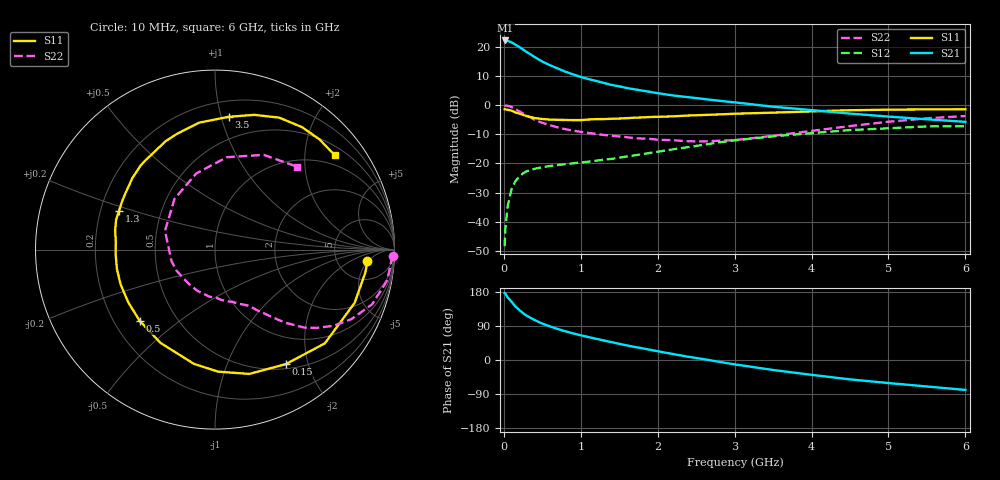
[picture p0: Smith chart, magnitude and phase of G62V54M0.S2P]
! SIEMENS Small Signal Semiconductors
! BFG193
! Si NPN RF Bipolar Junction Transistor in SOT223
! VCE = 2.5 V  IC = 4 mA
! Common Emitter S-Parameters:  August  1996
# GHz  S  MA  R  50
!  f  S11  S21  S12  S22
! GHz  MAG  ANG  MAG  ANG  MAG  ANG  MAG  ANG
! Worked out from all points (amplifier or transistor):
!   36 points, 10 MHz to 6 GHz, reference 50 ohm
!   highest |S21| = 22.2 dB at 20 MHz (marker M1)
!   |S21| within 3 dB of that: start of sweep to 243.1 MHz
!   unconditionally stable (mu >= 1): 1.209 GHz to 2.622 GHz
!   at 250 MHz: K = 0.29, MSG = 21.2 dB, |S12| = -23.4 dB
!   at 1.4 GHz: K = 1.09, MAG = 10.9 dB, |S12| = -18.4 dB
!   at 6 GHz: K = 0.92, MSG = 0.7 dB, |S12| = -7.2 dB
!   S11 on the Smith chart (normalised r, x): 10 MHz: 10, -5; 150 MHz: 0.56, -1.65; 500 MHz: 0.31, -0.37; 1.3 GHz: 0.28, +0.18; 3.5 GHz: 0.32, +1.06; 6 GHz: 0.72, +2.71
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0.01  0.851 -4.3  12.84 176.9  0.0038 89.4  0.9933 -2.0
0.02  0.8475 -8.6  12.9 175.1  0.0075 86.8  0.9831 -4.1
0.05  0.8326 -20.9  12.67 165.3  0.0186 78.9  0.9751 -10.1
0.1  0.8046 -40.5  11.95 153.8  0.036 70.3  0.927 -19.2
0.15  0.7502 -58.3  10.92 141.2  0.0493 60.3  0.8531 -27.0
0.2  0.7185 -74.6  9.979 132.2  0.0592 54.3  0.7855 -32.7
0.25  0.6801 -88.6  9 123.5  0.0676 48.5  0.7151 -37.6
0.3  0.6473 -100.5  8.134 116.5  0.0736 44.9  0.6593 -41.2
0.4  0.6018 -120.4  6.707 105.6  0.0808 39.0  0.5621 -46.3
0.5  0.5777 -136.6  5.592 96.0  0.086 35.3  0.4969 -49.5
0.6  0.5655 -148.8  4.848 88.6  0.0903 33.5  0.4518 -52.2
0.7  0.5605 -159.9  4.254 81.7  0.0936 32.7  0.416 -54.9
0.9  0.5542 -177.2  3.372 70.2  0.1005 32.1  0.3647 -59.1
1.1  0.5666 169.0  2.803 60.5  0.1072 32.6  0.3342 -65.2
1.3  0.5767 157.9  2.405 51.5  0.1162 33.2  0.3077 -71.2
1.6  0.5979 143.1  1.966 38.4  0.1316 33.5  0.2815 -83.3
2.2  0.6428 120.9  1.467 15.7  0.1745 30.9  0.2499 -113.3
2.8  0.6933 102.4  1.189 -4.8  0.2294 23.0  0.2454 -152.4
3.5  0.7439 84.1  0.941 -26.3  0.2918 8.3  0.2975 159.4
4.5  0.8178 64.0  0.717 -51.1  0.3737 -12.7  0.4372 103.8
5.5  0.8462 46.6  0.572 -69.9  0.4316 -38.7  0.5935 62.8
6  0.8496 38.3  0.517 -79.0  0.4357 -53.3  0.6505 45.2
